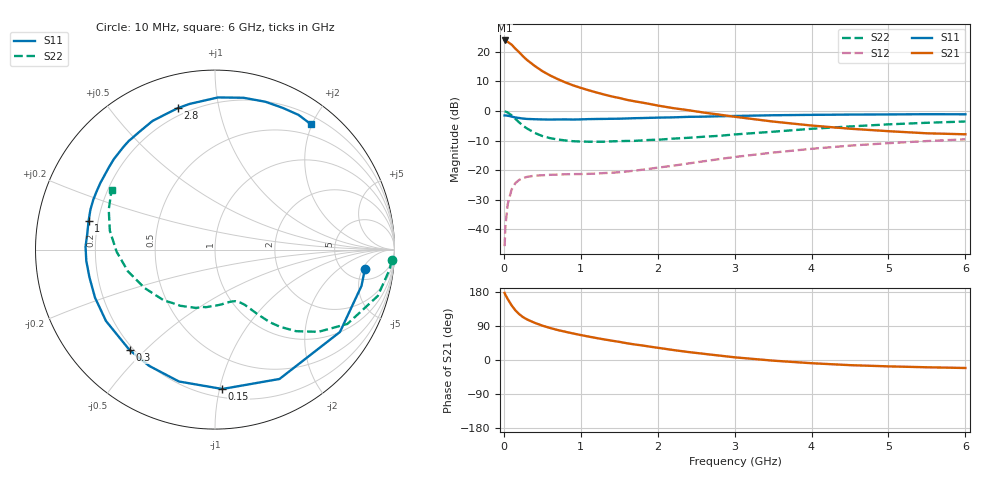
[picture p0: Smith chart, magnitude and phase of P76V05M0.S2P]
! SIEMENS Small Signal Semiconductors
! BFP196
! Si NPN RF Bipolar Junction Transistor in SOT143
! VCE = 6 V  IC = 5 mA
! Common Emitter S-Parameters:  May  1996
# GHz  S  MA  R  50
!  f  S11  S21  S12  S22
! GHz  MAG  ANG  MAG  ANG  MAG  ANG  MAG  ANG
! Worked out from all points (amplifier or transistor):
!   36 points, 10 MHz to 6 GHz, reference 50 ohm
!   highest |S21| = 23.8 dB at 10 MHz (marker M1)
!   |S21| within 3 dB of that: start of sweep to 159.5 MHz
!   unconditionally stable (mu >= 1): 1.148 GHz to 3.167 GHz
!   at 250 MHz: K = 0.25, MSG = 20.6 dB, |S12| = -22.7 dB
!   at 1.4 GHz: K = 1.15, MAG = 10.6 dB, |S12| = -20.9 dB
!   at 6 GHz: K = 0.99, MSG = 0.8 dB, |S12| = -9.6 dB
!   S11 on the Smith chart (normalised r, x): 10 MHz: 7.61, -5.52; 150 MHz: 0.26, -1.02; 300 MHz: 0.18, -0.45; 1 GHz: 0.16, +0.11; 2.8 GHz: 0.16, +0.76; 6 GHz: 0.32, +1.98
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0.01  0.842 -7.2  15.56 177.1  0.0052 90.1  0.9868 -3.4
0.02  0.841 -13.9  15.15 171.9  0.0111 80.2  0.979 -6.5
0.05  0.8338 -33.4  14.73 161.0  0.0265 73.1  0.9429 -15.9
0.1  0.8054 -63.5  13.27 144.4  0.0468 58.9  0.846 -29.3
0.15  0.7777 -87.0  11.32 131.0  0.0605 47.9  0.7359 -38.5
0.2  0.7618 -105.3  9.818 121.0  0.0686 40.1  0.6407 -45.2
0.25  0.7445 -119.6  8.395 113.1  0.0734 34.4  0.5618 -49.9
0.3  0.7347 -130.4  7.303 107.2  0.077 30.9  0.5078 -52.9
0.4  0.7261 -146.8  5.796 98.2  0.0808 26.1  0.4276 -56.8
0.5  0.72 -158.2  4.724 90.7  0.082 23.5  0.3777 -59.6
0.6  0.7164 -167.5  3.998 84.6  0.0835 22.1  0.3481 -61.8
0.7  0.7198 -175.0  3.463 79.1  0.0841 21.7  0.3302 -64.0
0.8  0.7214 178.8  3.04 74.5  0.0853 21.4  0.318 -66.2
1  0.7221 167.4  2.461 65.8  0.0861 23.1  0.3047 -71.2
1.1  0.7289 162.2  2.247 61.9  0.0867 24.2  0.3029 -74.0
1.6  0.7481 142.2  1.542 44.2  0.095 31.8  0.3119 -88.9
2.2  0.7805 122.3  1.119 26.4  0.119 38.9  0.3415 -107.9
2.8  0.8149 104.8  0.869 11.7  0.1539 39.7  0.3808 -128.7
3.5  0.8479 88.9  0.663 -1.7  0.1984 34.8  0.4466 -151.3
4.5  0.8703 71.2  0.502 -13.6  0.26 23.8  0.5484 -178.8
5.5  0.8831 58.2  0.42 -19.2  0.3107 11.2  0.6325 159.4
6  0.8793 52.6  0.404 -21.1  0.3323 4.5  0.665 150.0
